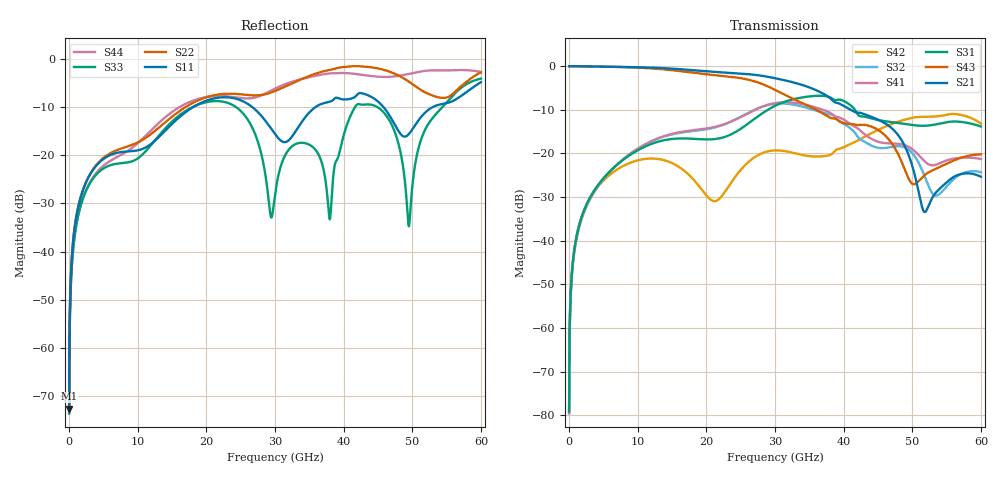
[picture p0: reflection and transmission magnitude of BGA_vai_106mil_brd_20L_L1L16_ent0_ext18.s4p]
# GHz S RI R 50
! S-Parameters data
! Freq  reS11  imS11  reS12  imS12  reS13  imS13  reS14  imS14
!  reS21  imS21  reS22  imS22  reS23  imS23  reS24  imS24
!  reS31  imS31  reS32  imS32  reS33  imS33  reS34  imS34
!  reS41  imS41  reS42  imS42  reS43  imS43  reS44  imS44
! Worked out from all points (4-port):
!   6000 points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, 10 MHz to 60 GHz, reference 50 ohm
!   strongest paths, dB at 10 MHz, 15.01 GHz, 30.01 GHz, 45.01 GHz, 60 GHz:
!     S21: 0.0, -0.6, -2.8, -12.2, -25.3
!     S43: 0.0, -0.9, -5.4, -14.6, -20.2
!     S31: -79.1, -16.7, -9.1, -12.3, -13.8
!     S41: -79.5, -15.5, -8.5, -17.3, -21.3
!     S32: -79.5, -15.6, -8.6, -18.7, -24.3
!     S42: -79.1, -22.2, -19.3, -14.6, -13.1
!   lowest |S11| = -72.7 dB at 10 MHz (marker M1), VSWR 1.00, Z = 50 - j0.0178 ohm
!   |S11| at or under -10 dB: start of sweep to 18.04 GHz; 26.73 GHz to 35.87 GHz (9.142 GHz wide, 29.2 % of centre); 45.83 GHz to 52.93 GHz (7.1 GHz wide, 14.4 % of centre)
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0.01  0.000149 -0.000178  0.9998 -0.00193  1.93e-05 0.000109  -1.93e-05 -0.000104
      0.9998 -0.00193  0.00015 -0.000178  -1.93e-05 -0.000104  1.94e-05 0.000109
      1.93e-05 0.000109  -1.93e-05 -0.000104  0.000158 -0.000135  0.9998 -0.00198
      -1.93e-05 -0.000104  1.94e-05 0.000109  0.9998 -0.00198  0.000158 -0.000135
2.18  -0.0211 -0.0415  0.9146 -0.3944  0.00761 0.021  -0.00839 -0.0196
      0.9146 -0.3944  -0.0126 -0.045  -0.00795 -0.0198  0.00924 0.0201
      0.00761 0.021  -0.00795 -0.0198  -0.0176 -0.0337  0.9093 -0.4052
      -0.00839 -0.0196  0.00924 0.0201  0.9093 -0.4052  -0.00864 -0.0375
11.82  0.0571 0.1161  -0.5734 -0.7739  0.1085 -0.0664  -0.096 0.0968
       -0.5734 -0.7739  -0.1189 -0.1129  -0.1051 0.0857  0.0534 -0.0693
       0.1085 -0.0664  -0.1051 0.0857  0.098 0.0773  -0.6198 -0.7135
       -0.096 0.0968  0.0534 -0.0693  -0.6198 -0.7135  -0.1031 -0.1453
24  -0.2675 -0.2882  -0.1297 0.8228  -0.0605 0.1606  0.2386 -0.0189
    -0.1297 0.8228  -0.4029 0.1689  0.2374 0.0365  0.0513 0.00245
    -0.0605 0.1606  0.2374 0.0365  -0.2669 -0.1918  -0.0047 0.7478
    0.2386 -0.0189  0.0513 0.00245  -0.0047 0.7478  -0.3716 0.1565
44.98  -0.3436 -0.1213  -0.2266 -0.0926  0.2267 0.0845  0.0606 0.1224
       -0.2266 -0.0926  0.6166 0.5132  0.0111 0.1158  0.00586 -0.1854
       0.2267 0.0845  0.0111 0.1158  -0.1512 -0.2769  -0.1361 -0.1283
       0.0606 0.1224  0.00586 -0.1854  -0.1361 -0.1283  0.3977 0.5241
49.51  0.1089 0.1262  -0.0495 0.0803  0.00334 -0.2147  0.1139 0.034
       -0.0495 0.0803  0.5784 0.0749  0.099 0.0486  -0.2392 -0.0761
       0.00334 -0.2147  0.099 0.0486  -0.000498 0.0183  -0.0508 -0.00225
       0.1139 0.034  -0.2392 -0.0761  -0.0508 -0.00225  0.5762 0.4038
60  0.3111 -0.4859  -0.0166 0.0516  0.2034 0.0107  0.0242 -0.083
    -0.0166 0.0516  0.7266 -0.0373  0.0467 -0.0395  0.2005 0.0932
    0.2034 0.0107  0.0467 -0.0395  0.2277 -0.585  -0.0735 0.0644
    0.0242 -0.083  0.2005 0.0932  -0.0735 0.0644  0.6302 -0.3842
